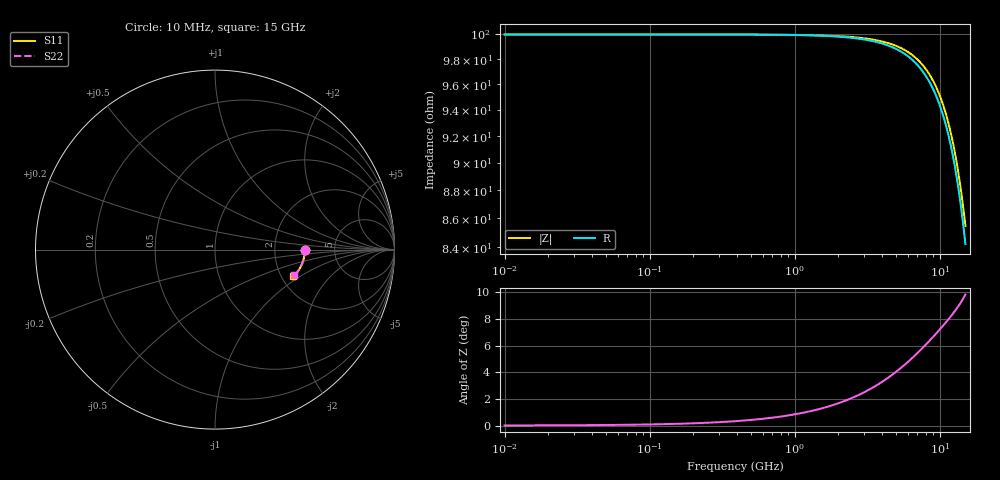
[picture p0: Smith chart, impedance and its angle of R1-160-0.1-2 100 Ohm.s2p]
!version-2
!date-03.2021
# MHz S RI R 50
!Freq ReS11 ImS11 ReS21 ImS21 ReS12 ImS12 ReS22 ImS22
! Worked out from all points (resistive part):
!   751 points, 10 MHz to 15 GHz, reference 50 ohm
!   read as one part in series: R = 100 ohm at 70 MHz
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10  0.5 -8.78e-05  0.5 -0.00011  0.5 -0.00011  0.5 -8.23e-05
70  0.5 -0.000615  0.5 -0.00077  0.5 -0.00077  0.5 -0.000576
1270  0.4997 -0.0112  0.4999 -0.014  0.4999 -0.014  0.4998 -0.0105
2510  0.4989 -0.0222  0.4998 -0.0275  0.4998 -0.0275  0.4991 -0.0208
3790  0.4975 -0.0338  0.4996 -0.0415  0.4996 -0.0415  0.4978 -0.0317
5010  0.4955 -0.0451  0.4994 -0.0546  0.4994 -0.0546  0.4961 -0.0423
6290  0.4926 -0.0573  0.4993 -0.0683  0.4993 -0.0683  0.4935 -0.0539
6910  0.4908 -0.0634  0.4993 -0.0749  0.4993 -0.0749  0.4919 -0.0597
7510  0.4889 -0.0694  0.4993 -0.0812  0.4993 -0.0812  0.4902 -0.0653
8150  0.4866 -0.0758  0.4995 -0.0879  0.4995 -0.0879  0.4881 -0.0715
8790  0.4839 -0.0824  0.4998 -0.0947  0.4998 -0.0947  0.4858 -0.0777
9410  0.4811 -0.0889  0.5001 -0.1012  0.5001 -0.1012  0.4832 -0.0839
10010  0.478 -0.0952  0.5006 -0.1075  0.5006 -0.1075  0.4804 -0.0899
10650  0.4743 -0.1021  0.5013 -0.1143  0.5013 -0.1143  0.477 -0.0965
11290  0.4702 -0.109  0.5021 -0.1211  0.5021 -0.1211  0.4733 -0.1031
11910  0.4658 -0.1157  0.5031 -0.1278  0.5031 -0.1278  0.4693 -0.1096
12510  0.4611 -0.1223  0.5043 -0.1344  0.5043 -0.1344  0.465 -0.1159
13130  0.4559 -0.129  0.5056 -0.1414  0.5056 -0.1414  0.4602 -0.1224
13730  0.4503 -0.1356  0.5072 -0.1482  0.5072 -0.1482  0.4551 -0.1287
14290  0.4447 -0.1416  0.5088 -0.1548  0.5088 -0.1548  0.4499 -0.1346
14930  0.4378 -0.1485  0.5109 -0.1626  0.5109 -0.1626  0.4435 -0.1412
15000  0.437 -0.1492  0.5112 -0.1635  0.5112 -0.1635  0.4428 -0.142
